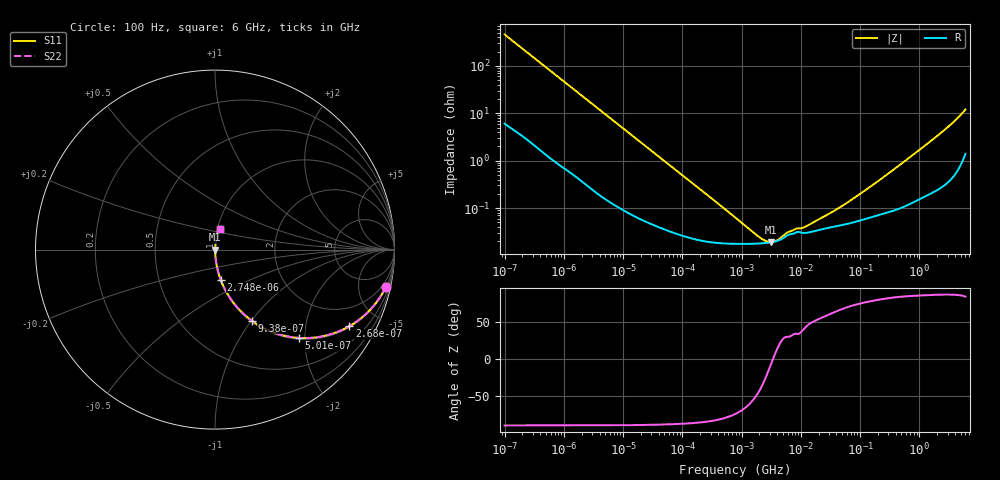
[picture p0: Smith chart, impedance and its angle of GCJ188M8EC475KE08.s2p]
!Murata Part Number: GCJ188M8EC475KE08
!These Parameters are Measured in Series Mode Connection
!Data Generated on Mar 13, 2026
!  o--ll--o
!Port1  Port2
!  o------o
!Operation Temp=25[degC], DC Bias Voltage=0[V]
!Freq. Start=100[Hz] Stop=6[GHz] 401[Steps]
# Hz S RI R 50
!Freq.(Hz) S11(Real) S11(Imag) S21(Real) S21(Imag) S12(Real) S12(Imag) S22(Real) S22(Imag)
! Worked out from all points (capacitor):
!   401 points, 100 Hz to 6 GHz, reference 50 ohm
!   read as one part in series: C = 3.44 uF near 109 Hz
!   lowest |Z| = 19.1 mohm at 3.104 MHz (marker M1)
!   series resonance near 3.4 MHz, so ESL is about 640 pH
!   S11 on the Smith chart (normalised r, x): 100 Hz: 1.12, -9.22; 268 Hz: 1.05, -3.47; 501 Hz: 1.03, -1.87; 938 Hz: 1.01, -1.00; 2.748 kHz: 1.01, -0.35; 6 GHz: 1.03, +0.24
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100  0.9526 -0.2059  0.0474 0.2059  0.0474 0.2059  0.9526 -0.2059
164  0.8856 -0.3114  0.1144 0.3114  0.1144 0.3114  0.8856 -0.3114
268  0.7481 -0.427  0.2519 0.427  0.2519 0.427  0.7481 -0.427
366  0.6171 -0.4791  0.3829 0.4791  0.3829 0.4791  0.6171 -0.4791
501  0.4662 -0.4919  0.5338 0.4919  0.5338 0.4919  0.4662 -0.4919
938  0.2044 -0.396  0.7956 0.396  0.7956 0.396  0.2044 -0.396
1342  0.1137 -0.31  0.8863 0.31  0.8863 0.31  0.1137 -0.31
2008  0.0558 -0.222  0.9442 0.222  0.9442 0.222  0.0558 -0.222
2748  0.0315 -0.1671  0.9685 0.1671  0.9685 0.1671  0.0315 -0.1671
8047  0.00459 -0.0593  0.9954 0.0593  0.9954 0.0593  0.00459 -0.0593
40335  0.000539 -0.0121  0.9995 0.0121  0.9995 0.0121  0.000539 -0.0121
774597  0.000176 -0.000615  0.9998 0.000615  0.9998 0.000615  0.000176 -0.000615
2074311  0.000179 -0.000152  0.9998 0.000152  0.9998 0.000152  0.000179 -0.000152
3103719  0.000189 -2.72e-05  0.9998 2.72e-05  0.9998 2.72e-05  0.000189 -2.72e-05
4060267  0.000204 5.32e-05  0.9998 -5.32e-05  0.9998 -5.32e-05  0.000204 5.32e-05
6353432  0.000276 0.000157  0.9997 -0.000157  0.9997 -0.000157  0.000276 0.000157
1.137099e7  0.000298 0.000255  0.9997 -0.000255  0.9997 -0.000255  0.000298 0.000255
1.555665e7  0.000318 0.000366  0.9997 -0.000366  0.9997 -0.000366  0.000318 0.000366
5.449875e7  0.00045 0.0011  0.9996 -0.0011  0.9996 -0.0011  0.00045 0.0011
3.124326e8  0.000854 0.00548  0.9991 -0.00548  0.9991 -0.00548  0.000854 0.00548
2.240541e9  0.00396 0.0369  0.996 -0.0369  0.996 -0.0369  0.00396 0.0369
6e9  0.0274 0.1151  0.9726 -0.1151  0.9726 -0.1151  0.0274 0.1151
